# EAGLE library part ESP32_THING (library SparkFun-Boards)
SparkFun ESP32 Thing Board Pins, silkscreen, and logos matching the layout of the SparkFun ESP32 Thing Dimensions: 2.32" x 1.00"
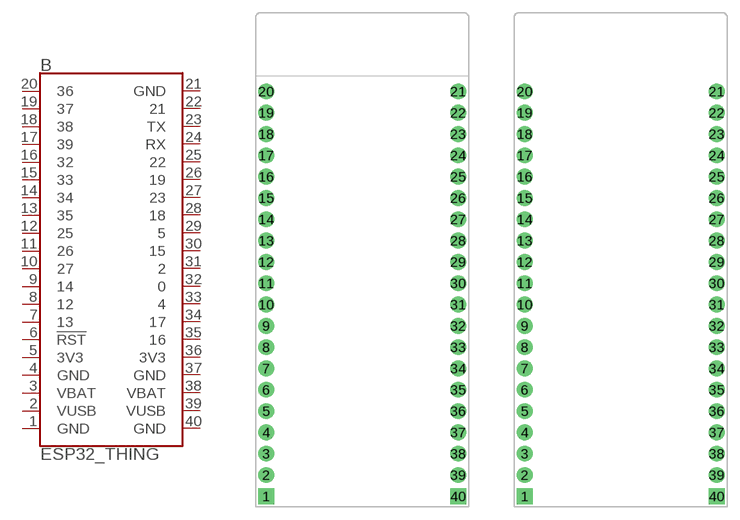
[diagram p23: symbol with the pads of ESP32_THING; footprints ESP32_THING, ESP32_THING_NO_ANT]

Designator prefix B

## ESP32_THING_W_ANT_KEEPOUT (SF_ID: DEV-13907)  [ESP32_THING]
1  GND
2  VUSB
3  VBAT
4  GND
5  3V3
6  !RST!
7  13
8  12
9  14
10  27
11  26
12  25
13  35
14  34
15  33
16  32
17  39
18  38
19  37
20  36
21  GND
22  21
23  TX
24  RX
25  22
26  19
27  23
28  18
29  5
30  15
31  2
32  0
33  4
34  17
35  16
36  3V3
37  GND
38  VBAT
39  VUSB
40  GND

## ESP32_THING_WO_ANT_KEEPOUT  [ESP32_THING_NO_ANT]
Pads as for ESP32_THING

## Footprint ESP32_THING (pad centres in mm)
SparkFun ESP32 Thing Board Pins, silkscreen, and logos matching the layout of the SparkFun ESP32 Thing Specifications: Pin count: 40 Area: 2.32" x 1.00"
drill 1.016 pad 1.88 square: 1 1.27,1.27; 40 24.13,1.27
drill 1.016 pad 1.88: 2 1.27,3.81; 3 1.27,6.35; 4 1.27,8.89; 5 1.27,11.43; 6 1.27,13.97; 7 1.27,16.51; 8 1.27,19.05; 9 1.27,21.59; 10 1.27,24.13; 11 1.27,26.67; 12 1.27,29.21; 13 1.27,31.75; 14 1.27,34.29; 15 1.27,36.83; 16 1.27,39.37; 17 1.27,41.91; 18 1.27,44.45; 19 1.27,46.99; 20 1.27,49.53; 21 24.13,49.53; 22 24.13,46.99; 23 24.13,44.45; 24 24.13,41.91; 25 24.13,39.37; 26 24.13,36.83; 27 24.13,34.29; 28 24.13,31.75; 29 24.13,29.21; 30 24.13,26.67; 31 24.13,24.13; 32 24.13,21.59; 33 24.13,19.05; 34 24.13,16.51; 35 24.13,13.97; 36 24.13,11.43; 37 24.13,8.89; 38 24.13,6.35; 39 24.13,3.81

## Footprint ESP32_THING_NO_ANT (pad centres in mm)
drill 1.016 pad 1.88 square: 1 1.27,1.27; 40 24.13,1.27
drill 1.016 pad 1.88: 2 1.27,3.81; 3 1.27,6.35; 4 1.27,8.89; 5 1.27,11.43; 6 1.27,13.97; 7 1.27,16.51; 8 1.27,19.05; 9 1.27,21.59; 10 1.27,24.13; 11 1.27,26.67; 12 1.27,29.21; 13 1.27,31.75; 14 1.27,34.29; 15 1.27,36.83; 16 1.27,39.37; 17 1.27,41.91; 18 1.27,44.45; 19 1.27,46.99; 20 1.27,49.53; 21 24.13,49.53; 22 24.13,46.99; 23 24.13,44.45; 24 24.13,41.91; 25 24.13,39.37; 26 24.13,36.83; 27 24.13,34.29; 28 24.13,31.75; 29 24.13,29.21; 30 24.13,26.67; 31 24.13,24.13; 32 24.13,21.59; 33 24.13,19.05; 34 24.13,16.51; 35 24.13,13.97; 36 24.13,11.43; 37 24.13,8.89; 38 24.13,6.35; 39 24.13,3.81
